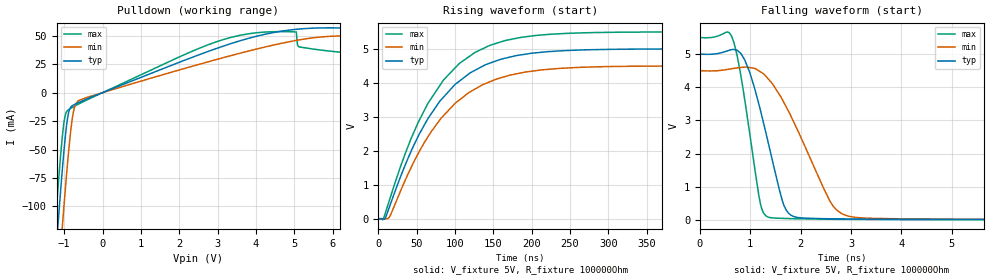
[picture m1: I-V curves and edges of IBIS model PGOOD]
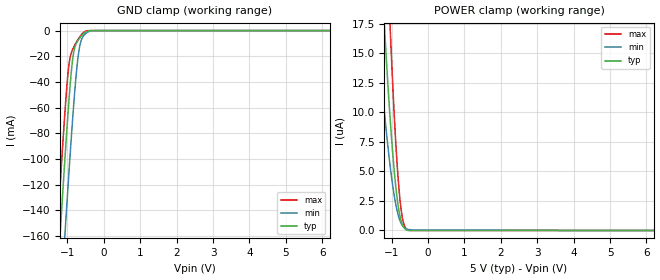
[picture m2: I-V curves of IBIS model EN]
|Texas Instruments Incorporated
| High Performance Single-Synchronous Step-Down Controller
| with Differential Voltage Feedback
| Marketing part#   Digital Voltage Range   Package-type   #pins
| TPS51219RTER   4.5V - 5.5V   WQFN   16
| TPS51219RTET   4.5V - 5.5V   WQFN   16
[IBIS Ver]   4.1
[File name]   tps51219.ibs
[File Rev]   1.0
[Date]   7/5/2012
[Source]
| Texas Instruments Incorporated.
| Analog-eLab Design Center, HPA
| 12500 TI Blvd
| Dallas, TX -75243
| e-mail: elab_scm_ibis@list.ti.com
[Notes]   Revision History:
| Rev 1.0: 7/5/2012
| - Initial version of the model
| - Model generated from simulations in TISPICE
| - C_comp although listed in numerical order of value are
|   obtained from varying PVT conditions. For PVT conditions for
|   each specific value refer the buffer description under
|   respective [Model]. IBIS model user is responsible for using
|   appropriate C_comp to simulate for Signal Integrity.
|  - Combined Non-monotonicity warnings of pulldown for PGOOD are minor
|   and reflect SPICE transistor simulations and can be ignored.
[Disclaimer]
| This model is designed as an aid for customers of Texas Instruments.
| TI and its licensors and suppliers make no warranties, either expressed
| or implied, with respect to this  model, including the warranties of
| merchantability or fitness for a particular purpose. The model is
| provided solely on an "as is" basis. The entire risk as to its quality
| and performance is with the customer.
[Copyright]
 (C) Copyright 2012 Texas Instruments Incorporated.All rights reserved.
|   TPS51219
[Component]   TPS51219
[Manufacturer]   TI
[Package]
|   typ   min   max
R_pkg   0.067   0.027   0.083
L_pkg   0.937nH   0.593nH   1.143nH
C_pkg   0.144pF   0.126pF   0.200pF
[Pin]  signal_name   model_name   R_pin   L_pin   C_pin
1   VREF   NC   0.07831   1.07402nH   0.13524pF
2   REFIN   NC   0.08036   1.0985nH   0.15151pF
3   GSNS   NC   0.0738   1.00365nH   0.14768pF
4   VSNS   NC   0.07415   1.01392nH   0.13413pF
5   COMP   NC   0.07231   0.98618nH   0.13415pF
6   TRIP   NC   0.06092   0.81627nH   0.13767pF
7   GND   GND   0.03163   0.59256nH   0.16679pF
8   PGND   NC   0.08348   1.14271nH   0.14722pF
9   V5   POWER   0.02705   0.69042nH   0.19997pF
10   DL   NC   0.07448   1.00522nH   0.14788pF
11   DH   NC   0.07496   1.01199nH   0.14633pF
12   SW   NC   0.07584   1.03028nH   0.13513pF
13   BST   NC   0.07155   0.96941nH   0.13065pF
14   EN   EN   0.06417   0.85929nH   0.1362pF
15   MODE   NC   0.06053   0.80931nH   0.13456pF
16   PGOOD   PGOOD   0.06512   0.88224nH   0.12591pF
| Models and submodels in the file (2): PGOOD (Open_drain), EN (Input)
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|   PGOOD Model
[Model]   PGOOD
Model_type   Open_drain
Polarity   Non-Inverting
Vmeas = 2.5
Vref = 5
Cref = 1pF
Rref = 100000
|   typ   min   max
C_comp   0.195pF   0.179pF   0.217pF
[Voltage Range]   5   4.5   5.5
[Temperature Range]   27   125   -40
[Pullup Reference]   5   4.5   5.5
[Pulldown Reference]   -0   -0   -0
[Power Clamp Reference]   5   4.5   5.5
[GND Clamp Reference]   -0   -0   -0
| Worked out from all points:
|   slope of the pulldown table from 0 to 0.75 V, typ, clamps not added: 74.5 ohm
|   falling waveform, V_fixture 5V, R_fixture 100000Ohm: 20-80 % time 482ps typ, 825ps min, 326ps max; typ from 5 V to 0.004 V
|   rising waveform, V_fixture 5V, R_fixture 100000Ohm: 20-80 % time 77.7ns typ, 80.9ns min, 75.9ns max; typ from 0.004 V to 5 V
[Pulldown]
|   Voltage   I(typ)   I(min)   I(max)
-5V       -1.997A    -2.043A    -1.969A
-1.25V    -155.9mA   -208mA     -123.3mA
-1.16V    -115.3mA   -167mA     -83.1mA
-1.04V    -64.26mA   -114mA     -35.76mA
-980mV    -41.77mA   -88.73mA   -20.77mA
-800mV    -11.76mA   -25.37mA   -13.24mA
-650mV    -9.078mA   -7.66mA    -10.44mA
3.16V     41.06mA    30.88mA    46.8mA
5.05V     55.7mA     45.94mA    53.36mA
6.31V     56.79mA    50.03mA    35.21mA
6.4V      42.64mA    50.1mA     34.94mA
9.97V     32.99mA    50.8mA     28.32mA
[Ramp]
R_load = 100000
|   typ   min   max
dV/dt_r   2.99809/7.77413e-08   2.6961/8.09044e-08   3.29815/7.59114e-08
dV/dt_f   2.99773/4.82394e-10   2.69589/8.24581e-10   3.29789/3.25716e-10
[Falling Waveform]
V_fixture = 5V
V_fixture_min = 4.5V
V_fixture_max = 5.5V
R_fixture = 100000Ohm
C_fixture = 0F
|   Time   V(typ)   V(min)   V(max)
0s        5V         4.498V     5.5V
675.8ps   5.14V      4.571V     5.352V
892.6ps   4.82V      4.608V     3.6V
1.17ns    3.497V     4.498V     741mV
1.274ns   2.861V     4.395V     182.9mV
1.71ns    300.9mV    3.417V     39.74mV
2.649ns   29.86mV    405.8mV    16.66mV
3.252ns   19.6mV     54.34mV    11.69mV
9.156ns   4.97mV     7.271mV    3.627mV
500ns     3.704mV    4.379mV    3.509mV
[Rising Waveform]
V_fixture = 5V
V_fixture_min = 4.5V
V_fixture_max = 5.5V
R_fixture = 100000Ohm
C_fixture = 0F
|   Time   V(typ)   V(min)   V(max)
0s        3.704mV    4.379mV    3.509mV
6.573ns   -6.917mV   -558.8uV   -13.2mV
14.4ns    328.3mV    38.82mV    527.1mV
42.37ns   1.958V     1.481V     2.33V
64.87ns   2.948V     2.41V      3.397V
85.27ns   3.583V     3.038V     4.087V
126.1ns   4.37V      3.816V     4.895V
171.7ns   4.76V      4.227V     5.276V
236.7ns   4.942V     4.428V     5.448V
500ns     5.001V     4.498V     5.5V
|   EN Model
[Model]   EN
Model_type   Input
Vinl = 0.8
Vinh = 3.5
|   typ   min   max
C_comp   1.523pF   1.444pF   1.561pF
[Voltage Range]   5   4.5   5.5
[Temperature Range]   27   125   -40
[Power Clamp Reference]   5   4.5   5.5
[GND Clamp Reference]   -0   -0   -0
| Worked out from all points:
|   GND clamp passes 1 mA (typ) near -0.49 V on its own axis
[GND Clamp]
|   Voltage   I(typ)   I(min)   I(max)
-5V       -2.024A    -2.079A    -1.99A
-1.43V    -266.3mA   -326.7mA   -228.1mA
-1.25V    -181.6mA   -242.1mA   -143.5mA
-1.19V    -154mA     -214.3mA   -116mA
-1.07V    -100.3mA   -159.6mA   -64.04mA
-950mV    -51.22mA   -107mA     -24.67mA
-830mV    -17.25mA   -58.53mA   -13.07mA
-740mV    -9.141mA   -28.57mA   -8.413mA
-680mV    -6.512mA   -14.82mA   -5.686mA
-590mV    -3.363mA   -5.505mA   -2.343mA
-470mV    -681.9uA   -1.712mA   -195uA
9.97V     0A         0A         0A
[POWER Clamp]
|   Voltage   I(typ)   I(min)   I(max)
-5V       79.82uA    79.73uA    88.41uA
-1.4V     28.62uA    17.33uA    37.27uA
-1.37V    27.06uA    16.16uA    36.66uA
-1.19V    16.87uA    9.771uA    28.86uA
-1.04V    9.433uA    5.433uA    17.17uA
-920mV    4.765uA    2.794uA    9.294uA
-860mV    2.994uA    1.818uA    6.113uA
-800mV    1.669uA    1.093uA    3.571uA
-710mV    519.2nA    442.7nA    1.149uA
-650mV    187nA      231.7nA    405.2nA
-590mV    45.95nA    126.8nA    105nA
9.97V     0A         0A         0A
